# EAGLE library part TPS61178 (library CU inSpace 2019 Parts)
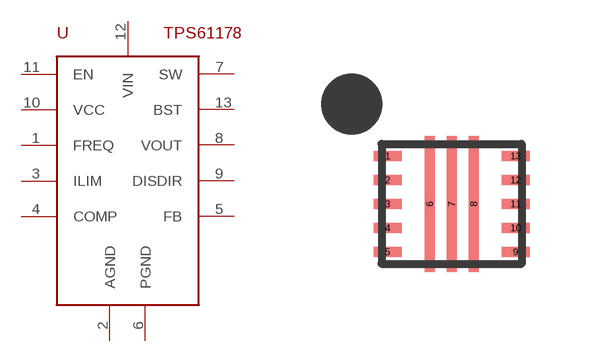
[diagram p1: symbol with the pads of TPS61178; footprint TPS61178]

Designator prefix U

## TPS61178  [TPS61178]
1  FREQ
2  AGND
3  ILIM
4  COMP
5  FB
6  PGND
7  SW
8  VOUT
9  DISDIR
10  VCC
11  EN
12  VIN
13  BST

## Footprint TPS61178 (pad centres in mm)
smd 0.7 x 0.25: 1 -1.6,1.2; 2 -1.6,0.6; 3 -1.6,0; 4 -1.6,-0.6; 5 -1.6,-1.2; 9 1.6,-1.2; 10 1.6,-0.6; 11 1.6,0; 12 1.6,0.6; 13 1.6,1.2
smd 0.25 x 3.4: 6 -0.55,0; 7 0,0; 8 0.55,0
